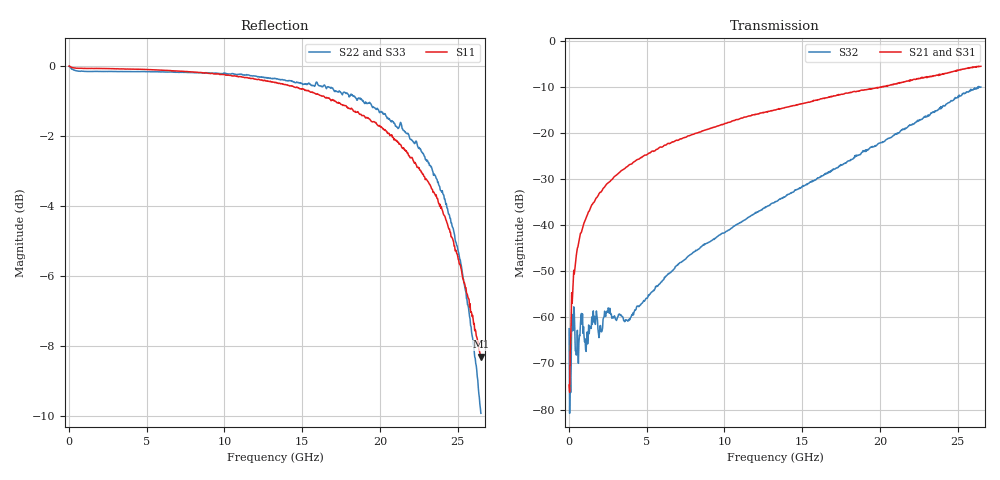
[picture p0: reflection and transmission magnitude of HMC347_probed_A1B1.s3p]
! Hittite Microwave Corporation
! 20 Alpha Road
! Chelmsford, MA 01824
! http://www.hittite.com
! Tel: 978-250-3343
! Fax: 978-250-3373
! Device:  HMC347
! Description: GaAs MMIC SPDT Non-Reflective Switch
! Frequency:  DC -  20.00 GHz
! Package:  DIE
! Ports:  3 RF, 2 DC
!  Pad  1 = RF1 = Port 2
!  Pad  2 = Control A [Alternate]
!  Pad  3 = Control B [Alternate]
!  Pad  4 = RFC = Port 1
!  Pad  5 = Control A [Alternate]
!  Pad  6 = Control B [Alternate]
!  Pad  7 = RF2 = Port 3
!  Pad  8 = Control A
!  Pad  9 = Control B
!  Pad 10 = Control A [Alternate]
! Control:  -5 Volt control voltage
!  Low  = 0 =  0 V
!  High = 1 = -5 V
! State:  Both High, Undefined
! Voltages:  VA = -5.0 Volts
!  VB = -5.0 Volts
! Data:  The device was measured using G-S-G Probes at the chip ports.
!  Data was collected using an calibrated 3 port network analyzer.
!  The reference plane is the pads on the switch chip.
! Misc:  Die 64601
!  Lot GB01, Tested Unit 3
! Date Measured:  2010-03-11
! Date:  2010-03-15
! Note:
!  Hittite supplies this data as a sample of measured data at the package pin for
!  for this package product.  Your particular data for this product may vary.
!  Data was taken at 25 degrees C.
!  Hittite reserves the right to change this data at anytime.
!S3P File: Measurements: <S11,S12,S13>,
!  <S21,S22,S23>,
!  <S31,S32,S33>:
# Hz S  dB  R 50
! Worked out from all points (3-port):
!   801 points, 10 MHz to 26.5 GHz, reference 50 ohm
!   strongest paths, dB at 10 MHz, 6.633 GHz, 13.26 GHz, 19.88 GHz, 26.5 GHz:
!     S21: -74.7, -22.0, -15.1, -10.3, -5.6
!     S31: -63.5, -22.2, -15.2, -10.0, -5.8
!     S32: -62.5, -50.0, -34.9, -22.4, -10.1
!   lowest |S11| = -8.3 dB at 26.5 GHz (marker M1), VSWR 2.25, Z = 26.5 - j19.2 ohm
!   |S11| at or under -10 dB: nowhere
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1e7  0.00 -0.0  -76.69 -122.6  -79.37 61.0
     -74.66 31.8  -0.00 -0.1  -76.53 -64.8
     -63.50 146.9  -62.46 33.4  -0.00 -0.0
2.749e8  -0.04 -1.2  -52.21 111.3  -52.59 114.6
         -52.62 112.4  -0.10 -2.1  -63.37 35.7
         -52.57 111.0  -62.67 34.0  -0.10 -2.2
5.729125e8  -0.06 -2.5  -44.19 104.8  -44.32 103.8
            -44.77 104.7  -0.14 -4.0  -66.69 30.7
            -44.32 103.9  -67.00 34.8  -0.13 -4.0
8.047e8  -0.06 -3.5  -40.84 96.0  -40.95 96.4
         -41.50 96.4  -0.14 -5.4  -59.03 26.9
         -40.98 96.0  -59.16 26.9  -0.14 -5.4
1.102712e9  -0.06 -4.8  -37.96 94.1  -38.13 93.5
            -38.43 94.3  -0.15 -7.3  -67.48 37.4
            -38.15 93.4  -67.39 36.9  -0.14 -7.3
2.096088e9  -0.06 -9.2  -32.16 83.9  -32.35 83.3
            -32.65 84.7  -0.15 -13.7  -63.73 51.8
            -32.38 83.2  -63.14 50.2  -0.15 -13.6
1.3255e10  -0.47 -59.9  -14.99 15.8  -15.17 14.8
           -15.07 17.0  -0.35 -87.3  -34.99 57.1
           -15.18 15.4  -34.93 56.0  -0.40 -86.9
2.176491e10  -2.48 -102.8  -8.62 -43.0  -8.74 -44.7
             -8.78 -43.3  -1.93 -153.5  -19.33 -30.6
             -8.69 -45.6  -18.82 -32.1  -1.94 -152.8
2.424835e10  -4.39 -116.8  -6.81 -65.0  -6.88 -67.5
             -7.08 -65.5  -3.94 177.0  -14.35 -72.1
             -6.89 -68.7  -13.80 -74.4  -3.72 176.9
2.65e10  -8.30 -126.8  -5.43 -90.1  -5.56 -93.2
         -5.56 -91.3  -9.91 130.4  -10.38 -129.1
         -5.76 -94.5  -10.05 -131.0  -9.36 129.6
